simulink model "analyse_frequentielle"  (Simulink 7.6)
settings: Solver=ode15s  SolverMode=SingleTasking  StartTime=0.0  StopTime=6e-3  RelTol=1e-3  AbsTol=1e-6
InitFcn:
  | clear all
  | close all
  | delete *.mat
StopFcn:
  | close all
  | load I_V.mat
  | plotyy(x(1,:),x(2,:),x(1,:),x(3,:))
  | title('Tension et courant de sortie')
  | grid
libraries: powerlib x11

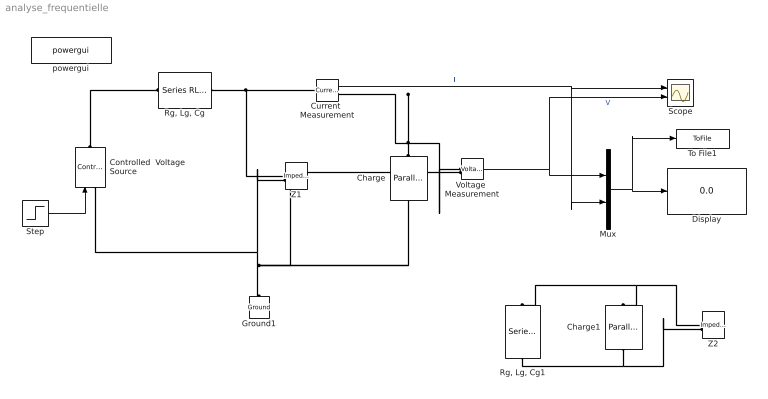
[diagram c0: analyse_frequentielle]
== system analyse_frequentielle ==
  Charge : powerlib/Elements/Parallel RLC Branch  DialogController=POWERSYS.PowerSysDialog  PhysicalDomain=powersysdomain  SubClassName=unknown  LeftPortType=p1  RightPortType=p1  LConnTagsString=a  RConnTagsString=__new0  BranchType=RLC  Resistance=1000  Inductance=1e-02  SetiL0=off  InitialCurrent=0  Capacitance=0  Setx0=off  InitialVoltage=0  Measurements=None
  Charge1 : powerlib/Elements/Parallel RLC Branch  DialogController=POWERSYS.PowerSysDialog  PhysicalDomain=powersysdomain  SubClassName=unknown  LeftPortType=p1  RightPortType=p1  LConnTagsString=a  RConnTagsString=__new0  BranchType=RLC  Resistance=1000  Inductance=1e-02  SetiL0=off  InitialCurrent=0  Capacitance=0  Setx0=off  InitialVoltage=0  Measurements=None
  Controlled  Voltage Source : powerlib/Electrical Sources/Controlled Voltage Source  DialogController=POWERSYS.PowerSysDialog  SystemSampleTime=-1  Initialize=on  Source_Type=AC  Amplitude=0  Phase=0  Frequency=0  Measurements=None
  Current  Measurement : powerlib/Measurements/Current Measurement  Tag=PoWeRsYsTeMmEaSuReMeNt  DialogController=POWERSYS.PowerSysDialog  SystemSampleTime=-1  PhasorSimulation=off  OutputType=Magnitude  PSBequivalent=0
  Display : Display
  Ground1 : powerlib/Elements/Ground  DialogController=POWERSYS.PowerSysDialog  PhysicalDomain=powersysdomain  SubClassName=unknown  LeftPortType=p1  RightPortType=p1  LConnTagsString=a
  Mux : Mux  Inputs=2
  "Rg, Lg, Cg" : powerlib/Elements/Series RLC Branch  DialogController=POWERSYS.PowerSysDialog  PhysicalDomain=powersysdomain  SubClassName=unknown  LeftPortType=p1  RightPortType=p1  LConnTagsString=__new0  RConnTagsString=__new0  BranchType=RLC  Resistance=47  Inductance=10e-03  SetiL0=off  InitialCurrent=0  Capacitance=1e-06  Setx0=off  InitialVoltage=0  Measurements=None
  "Rg, Lg, Cg1" : powerlib/Elements/Series RLC Branch  DialogController=POWERSYS.PowerSysDialog  PhysicalDomain=powersysdomain  SubClassName=unknown  LeftPortType=p1  RightPortType=p1  LConnTagsString=__new0  RConnTagsString=__new0  BranchType=RLC  Resistance=47  Inductance=10e-03  SetiL0=off  InitialCurrent=0  Capacitance=1e-06  Setx0=off  InitialVoltage=0  Measurements=None
  Scope : Scope  NumInputPorts=2
  Step : Step  Time=0  After=12  SampleTime=0
  To File1 : ToFile  Filename=I_V  MatrixName=x
  Voltage  Measurement : powerlib/Measurements/Voltage Measurement  Tag=PoWeRsYsTeMmEaSuReMeNt  DialogController=POWERSYS.PowerSysDialog  SystemSampleTime=-1  PhasorSimulation=off  OutputType=Magnitude  PSBequivalent=0
  Z1 : powerlib/Measurements/Impedance Measurement  DialogController=POWERSYS.PowerSysDialog  PhysicalDomain=powersysdomain  SubClassName=unknown  LeftPortType=p1  RightPortType=p1  LConnTagsString=+|-  Factor=1
  Z2 : powerlib/Measurements/Impedance Measurement  DialogController=POWERSYS.PowerSysDialog  PhysicalDomain=powersysdomain  SubClassName=unknown  LeftPortType=p1  RightPortType=p1  LConnTagsString=+|-  Factor=1
  powergui : powerlib/powergui  Priority=2  SystemSampleTime=-1  SimulationMode=Continuous  SampleTime=50e-6  frequency=60  SPID=off  DisableSnubberDevices=off  DisableRonSwitches=off  DisableVfSwitches=off  SwTol=0  Interpol=off  frequencyindice=60  echomessages=on  HookPort=off  DisplayEquations=off  FunctionMessages=off  EnableUseOfTLC=off  x0status=blocks  RestoreLinks=warning  ResistiveCurrentMeasurement=off  Frange=0:2:10000  Ylog=off  Xlog=off  ShowGrid=on  save=off  variable=ZData  ZoomFFT=on  StartTime=0.0  cycles=1  DisplayStyle=off  fundamental=60  FreqAxis=off  MaxFrequency=1000  frequencyindicesteady=1  RmsSteady=1  display=off  Ts=0  methode=off
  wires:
  Current  Measurement/1 -> Scope/1, Mux/2  "I"
  Voltage  Measurement/1 -> Scope/2, Mux/1  "V"
  Step/1 -> Controlled  Voltage Source/1
  Mux/1 -> Display/1, To File1/1
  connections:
  "Rg, Lg, Cg"/LConn1 -- Current  Measurement/LConn1 -- Z1/LConn1
  Controlled  Voltage Source/LConn1 -- Voltage  Measurement/LConn2 -- Charge/LConn1 -- Z1/LConn2 -- Ground1/LConn1
  Charge/RConn1 -- Current  Measurement/RConn1 -- Voltage  Measurement/LConn1
  Controlled  Voltage Source/RConn1 -- "Rg, Lg, Cg"/RConn1
  Z2/LConn1 -- Charge1/RConn1 -- "Rg, Lg, Cg1"/LConn1
  "Rg, Lg, Cg1"/RConn1 -- Charge1/LConn1 -- Z2/LConn2
